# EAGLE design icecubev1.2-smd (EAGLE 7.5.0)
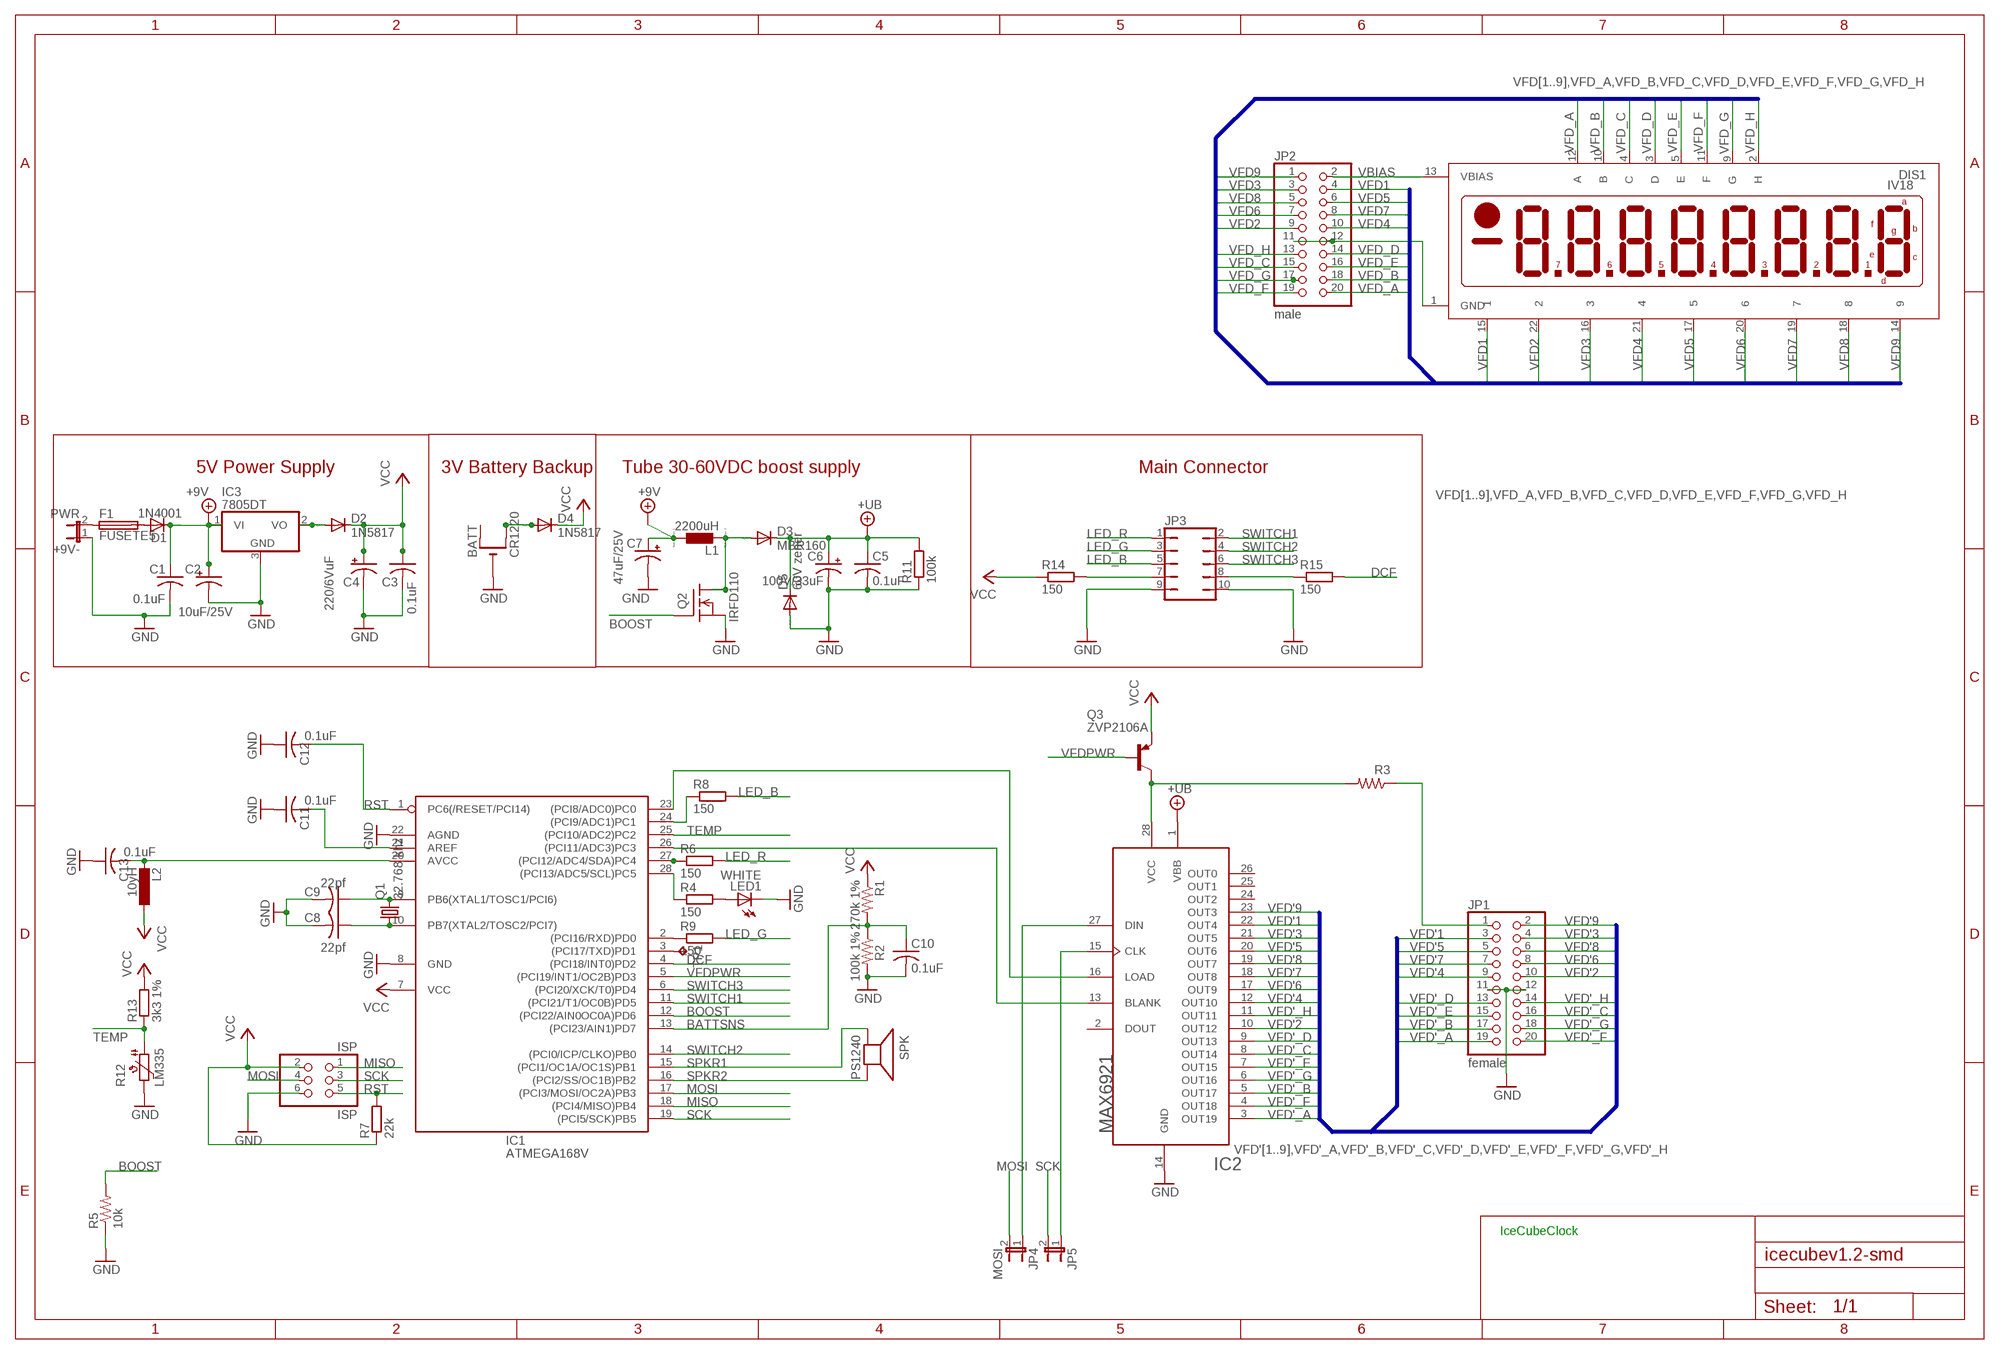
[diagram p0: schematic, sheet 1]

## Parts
+9V-  PWR  JP1E  [JP1]
BATT  CR1220  CR1220SMT  [CR1220-SMD]
C1  0.1uF  C-USC1206  [C1206]
C2  10uF/25V  CPOL-US153CLV-0405  [153CLV-0405]
C3  0.1uF  C-USC1206  [C1206]
C4  220/6VuF  CPOL-US153CLV-0405  [153CLV-0405]
C5  0.1uF  C-USC1206  [C1206]
C6  100V/33uF  CPOL-US153CLV-0405  [153CLV-0405]
C7  47uF/25V  CPOL-US153CLV-0405  [153CLV-0405]
C8  22pf  C-USC1206  [C1206]
C9  22pf  C-USC1206  [C1206]
C10  0.1uF  C-USC1206  [C1206]
C11  0.1uF  C-USC1206  [C1206]
C12  0.1uF  C-USC1206  [C1206]
C13  0.1uF  C-USC1206  [C1206]
D1  1N4001  DIODE-SOD80C  [SOD80C]
D2  1N5817  DIODE-SOD80C  [SOD80C]
D3  MBR160  DIODE-SOD80C  [SOD80C]
D4  1N5817  DIODE-SOD80C  [SOD80C]
D5  60V zener  DIODE-SOD80C  [SOD80C]
DIS1  IV18  [IV18]
F1  FUSETE5  [TE5]
IC1  ATMEGA168V  ATMEGA168PROUND  [DIL28/3]
IC2  MAX6921  [PLCC-S28]
IC3  7805DT  [TO252]
ISP  ISP  PINHD-2X3  [2X03]
JP1  female  PINHD-2X10  [2X10]
JP2  male  PINHD-2X10  [2X10]
JP3  JP5Q  [JP5Q]
JP4  MOSI  JP1E  [JP1]
JP5  JP1E  [JP1]
L1  2200uH  LL5650M  [L5650M]
L2  10yH  L-EUL4035M  [L4035M]
LED1  WHITE  LED5MM  [LED5MM]
Q1  32.768 khz  CRYTALTC26V  [TC26V]
Q2  IRFD110  [DIL04]
Q3  ZVP2106A  BC808-25-PNP-SOT23-BEC  [SOT23-BEC]
R1  270k 1%  R-US_M1206  [M1206]
R2  100k 1%  R-US_M1206  [M1206]
R3  22  R-US_M1206  [M1206]
R4  150  R-EU_M1206  [M1206]
R5  10k  R-US_R1206  [R1206]
R6  150  R-EU_M1206  [M1206]
R7  22k  R-EU_R1206  [R1206]
R8  150  R-EU_M1206  [M1206]
R9  150  R-EU_M1206  [M1206]
R11  100k  R-EU_R1206  [R1206]
R12  LM335  PTC-SOD70  [SOD70]
R13  3k3 1%  R-EU_M1206  [M1206]
R14  150  R-EU_R1206  [R1206]
R15  150  R-EU_R1206  [R1206]
SPK  PS1240  SPEAKER/PS12  [PS12]
TP1  TPB2,54  [B2,54]

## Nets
+9V: C1.1 C2.+ C7.+ D1.C IC3.1(VI) L1.1
+UB: C5.1 C6.+ D3.C D5.C IC2.1(VBB) R11.2
BATTSNS: C10.1 IC1.13((PCI23/AIN1)PD7) R1.2 R2.1
BLANK: IC1.26((PCI11/ADC3)PC3) IC2.13(BLANK)
BOOST: IC1.12((PCI22/AIN0OC0A)PD6) Q2.3(G) R5.2
DCF: IC1.4((PCI18/INT0)PD2) R15.2
GND: +9V-.1 BATT.- C1.2 C2.- C3.2 C4.- C5.2 C6.- C7.- C8.2 C9.2 C10.2 C11.1 C12.1 C13.1 D5.A DIS1.1(GND) IC1.8(GND) IC1.22(AGND) IC2.14(GND) IC3.3(GND) ISP.6 JP1.11 JP1.12 JP2.11 JP2.12 JP3.9 JP3.10 LED1.K(C) Q2.4(S) R2.2 R5.1 R11.1 R12.2
LED_B: JP3.5 R8.2
LED_G: JP3.3 R9.2
LED_R: JP3.1 R6.2
LOAD: IC1.23((PCI8/ADC0)PC0) IC2.16(LOAD)
MISO: IC1.18((PCI4/MISO)PB4) ISP.1
MOSI: IC1.17((PCI3/MOSI/OC2A)PB3) ISP.4 JP4.2
N$1: C9.1 IC1.9(PB6(XTAL1/TOSC1/PCI6)) Q1.2
N$2: D3.A L1.2 Q2.1(D) Q2.2(D1)
N$3: C8.1 IC1.10(PB7(XTAL2/TOSC2/PCI7)) Q1.1
N$4: +9V-.2 F1.1
N$5: D1.A F1.2
N$6: IC1.27((PCI12/ADC4/SDA)PC4) R6.1
N$7: IC1.28((PCI13/ADC5/SCL)PC5) R4.1
N$8: IC1.24((PCI9/ADC1)PC1) R8.1
N$9: IC1.2((PCI16/RXD)PD0) R9.1
N$10: BATT.+$2(+1) D4.A
N$11: JP3.8 R15.1
N$12: JP3.7 R14.2
N$13: LED1.A R4.2
N$14: C11.2 IC1.21(AREF)
N$15: C13.2 IC1.20(AVCC) L2.2
N$16: IC2.27(DIN) JP4.1
N$17: IC2.15(CLK) JP5.1
N$18: IC1.3((PCI17/TXD)PD1) TP1.TP
N$34: JP1.1 R3.1
N$39: IC2.28(VCC) Q3.C R3.2
N$53: D2.A IC3.2(VO)
RST: C12.2 IC1.1(PC6(/RESET/PCI14)) ISP.5 R7.2
SCK: IC1.19((PCI5/SCK)PB5) ISP.3 JP5.2
SPKR1: IC1.15((PCI1/OC1A/OC1S)PB1) SPK.P$1(+)
SPKR2: IC1.16((PCI2/SS/OC1B)PB2) SPK.P$2(-)
SWITCH1: IC1.11((PCI21/T1/OC0B)PD5) JP3.2
SWITCH2: IC1.14((PCI0/ICP/CLKO)PB0) JP3.4
SWITCH3: IC1.6((PCI20/XCK/T0)PD4) JP3.6
TEMP: IC1.25((PCI10/ADC2)PC2) R12.1 R13.1
VBIAS: DIS1.13(VBIAS) JP2.2
VCC: C3.1 C4.+ D2.C D4.C IC1.7(VCC) ISP.2 L2.1 Q3.E R1.1 R7.1 R13.2 R14.1
VFD1: DIS1.15 JP2.4
VFD2: DIS1.22 JP2.9
VFD3: DIS1.16 JP2.3
VFD4: DIS1.21 JP2.10
VFD5: DIS1.17 JP2.6
VFD6: DIS1.20 JP2.7
VFD7: DIS1.19 JP2.8
VFD8: DIS1.18 JP2.5
VFD9: DIS1.14 JP2.1
VFD'1: IC2.22(OUT4) JP1.3
VFD'2: IC2.10(OUT12) JP1.10
VFD'3: IC2.21(OUT5) JP1.4
VFD'4: IC2.12(OUT10) JP1.9
VFD'5: IC2.20(OUT6) JP1.5
VFD'6: IC2.17(OUT9) JP1.8
VFD'7: IC2.18(OUT8) JP1.7
VFD'8: IC2.19(OUT7) JP1.6
VFD'9: IC2.23(OUT3) JP1.2
VFD'_A: IC2.3(OUT19) JP1.19
VFD'_B: IC2.5(OUT17) JP1.17
VFD'_C: IC2.8(OUT14) JP1.16
VFD'_D: IC2.9(OUT13) JP1.13
VFD'_E: IC2.7(OUT15) JP1.15
VFD'_F: IC2.4(OUT18) JP1.20
VFD'_G: IC2.6(OUT16) JP1.18
VFD'_H: IC2.11(OUT11) JP1.14
VFD_A: DIS1.12(A) JP2.20
VFD_B: DIS1.10(B) JP2.18
VFD_C: DIS1.4(C) JP2.15
VFD_D: DIS1.3(D) JP2.14
VFD_E: DIS1.5(E) JP2.16
VFD_F: DIS1.11(F) JP2.19
VFD_G: DIS1.9(G) JP2.17
VFD_H: DIS1.2(H) JP2.13
VFDPWR: IC1.5((PCI19/INT1/OC2B)PD3) Q3.B
Unconnected: BATT.+$1(+) IC2.2(DOUT) IC2.24(OUT2) IC2.25(OUT1) IC2.26(OUT0)

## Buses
VFD[1..9],VFD_A,VFD_B,VFD_C,VFD_D,VFD_E,VFD_F,VFD_G,VFD_H
VFD'[1..9],VFD'_A,VFD'_B,VFD'_C,VFD'_D,VFD'_E,VFD'_F,VFD'_G,VFD'_H

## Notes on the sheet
- 5V Power Supply | 3V Battery Backup | Tube 30-60VDC boost supply | Main Connector
- IceCubeClock

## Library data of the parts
+9V- JP4 JP5 = jumper:JP1E: JUMPER
BATT = vfd:CR1220
C1 C3 C8 C9 C11-C13 = minimidi:C-US: CAPACITOR, American symbol
C2 C4 C7 = minimidi:CPOL-US: POLARIZED CAPACITOR, American symbol
C5 C10 = rcl-ez:C-US: CAPACITOR, American symbol
C6 = rcl-ez:CPOL-US: POLARIZED CAPACITOR, American symbol
D1-D5 = diode:DIODE-: DIODE
DIS1 = vfd:IV18: LCD DISPLAY 8-character 7 segment
F1 = fuse:FUSE: Fuse
IC1 = avr:ATMEGA168*P: MICROCONTROLLER 16 kBytes FLASH 1 kBytes SRAM 512 Bytes EEPROM USART 8-channel 10 bit ADC
IC2 = vfd:MAX6921
IC3 = linear:78*: Positive VOLTAGE REGULATOR
ISP = pinhead-ez:PINHD-2X3: PIN HEADER
JP1 JP2 = pinhead:PINHD-2X10: PIN HEADER
JP3 = jumper:JP5Q: JUMPER
L1 = eagle-ltspice:L: INDUCTOR, European symbol; SPICEMODEL: NONE; SPICEPREFIX: L
L2 = rcl:L-EU: INDUCTOR, European symbol
LED1 = led:LED: LED
Q1 = crystal:CRYTAL: CRYSTAL
Q2 = vfd:IRFD110
Q3 = transistor:*-PNP-: PNP Transistror
R1-R3 R5 = minimidi:R-US_: RESISTOR, American symbol
R4 R6 R8 R9 R13-R15 = resistor:R-EU_: RESISTOR, European symbol
R7 R11 = rcl:R-EU_: RESISTOR, European symbol
R12 = ptc-ntc:PTC-: Positive Temperature Coefficient Resistor (PTC) termistor; OC_FARNELL: unknown; OC_NEWARK: unknown
SPK = ybox2:SPEAKER: SPEAKER
TP1 = testpad:TP: Test pad

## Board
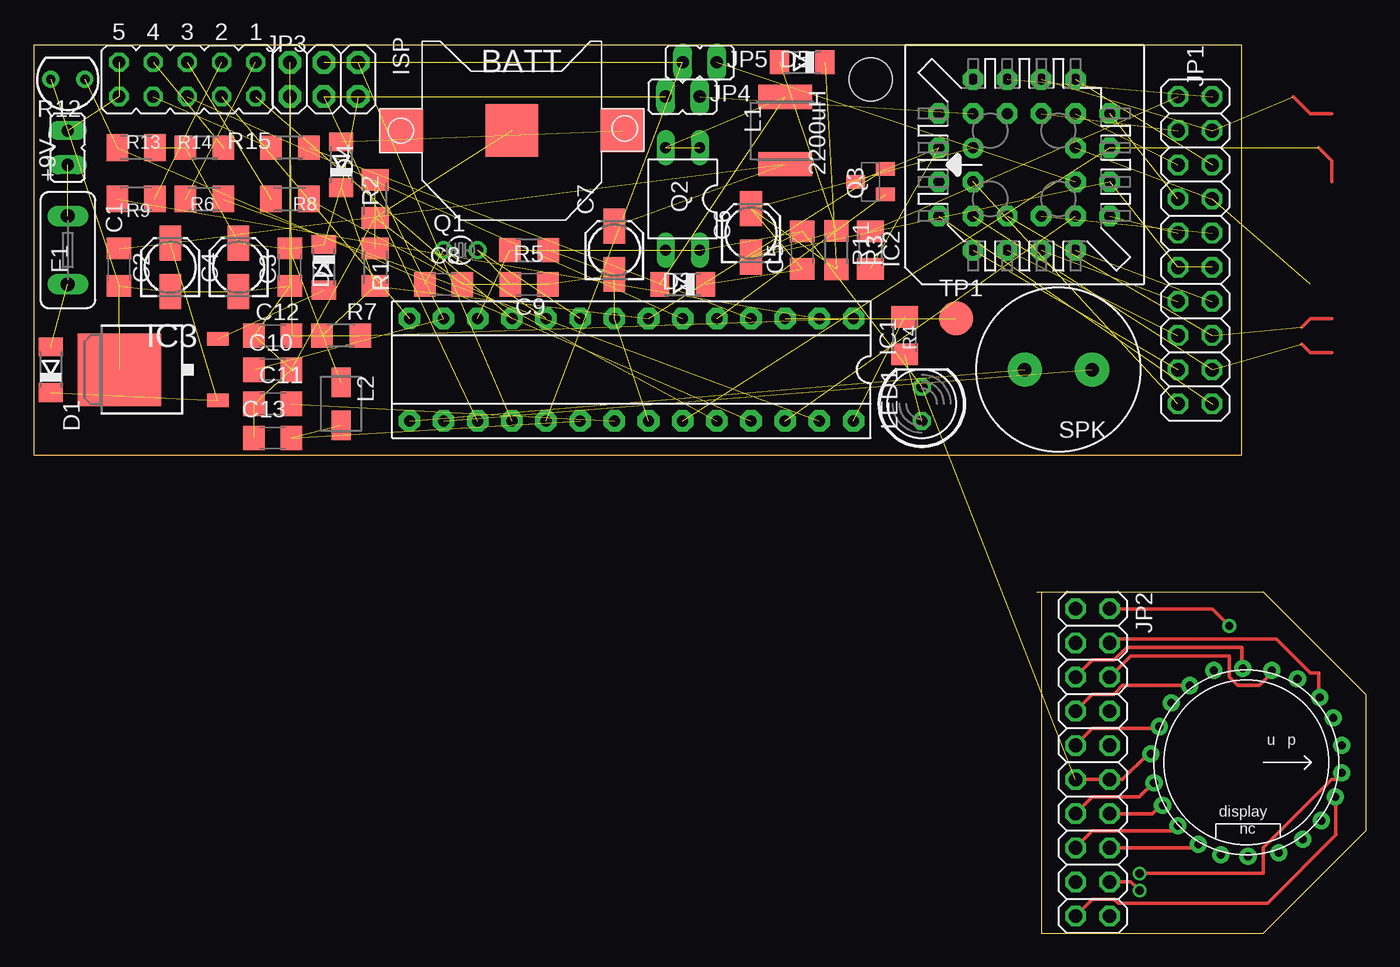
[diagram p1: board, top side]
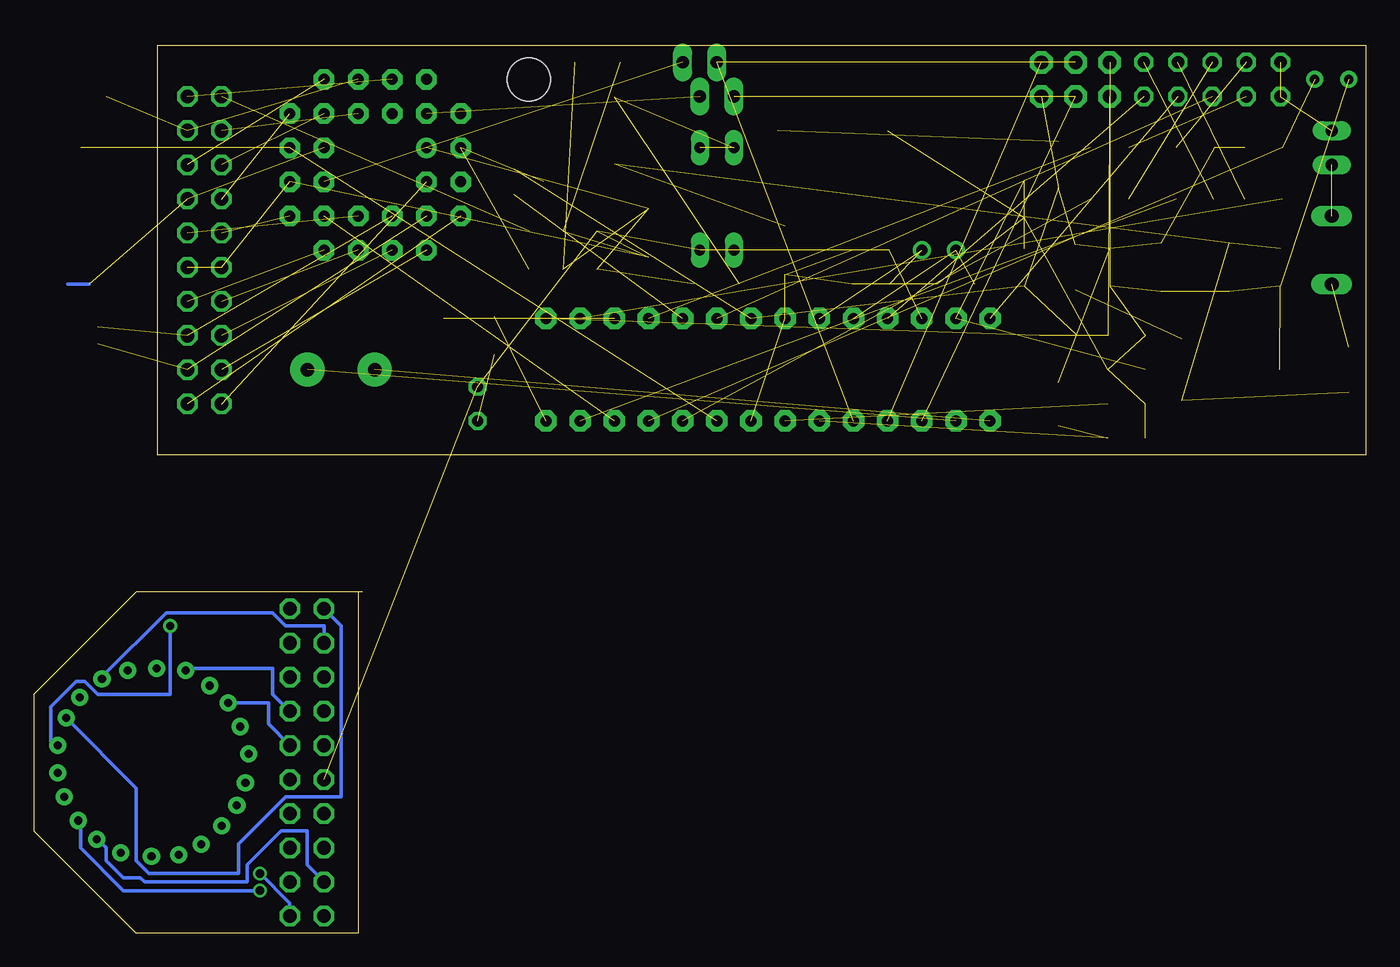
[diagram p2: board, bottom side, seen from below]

Size 99.06 x 66.03 mm. Coordinates in mm from the lower left corner, seen from the top.
Outline: 74.6,25.4 91.44,25.4 99.06,17.77 99.06,7.62
Outline: 74.93,25.39 74.93,0 91.44,0 99.06,7.61
Outline: 89.84,35.56 89.84,66.03 0,66.03 0,35.56 89.84,35.56
Copper layers (1*16): Top 0.035mm / dielectric 1.5mm / Bottom 0.035mm
Design rules "default": minimum track width 10mil, minimum drill 24mil, track to track 8mil, track to pad 8mil, pad to pad 8mil, via to via 8mil, smd to smd 8mil, copper to edge 40mil, drill to drill 8mil, minimum pad ring 10mil, minimum via ring 8mil, stop-mask expansion 4mil, vias tented up to drill 0mil, thermal gap 10mil
Holes 3.2 mm at 62.23,63.5

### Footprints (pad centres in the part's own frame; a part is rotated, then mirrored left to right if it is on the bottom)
JP1 = drill 0.914 long: 1 0,-1.27; 2 0,1.27
CR1220-SMD = smd 3.2 x 3.2: +$1 -8.2,0; +$2 8.2,0 | smd 3.9 x 3.9: - 0,0
C1206 = smd 1.6 x 1.8: 1 -1.4,0; 2 1.4,0
153CLV-0405 = smd 2.6 x 1.6: + 1.8,0; - -1.8,0
SOD80C = smd 1.4 x 1.8: A 1.7,0; C -1.7,0
IV18 = drill 0.6 pad 1.27: 1 -0.635,-7.112; 2 1.524,-6.858; 3 3.175,-6.223; 4 4.699,-5.08; 5 6.096,-3.556; 6 6.858,-1.905; 7 6.985,0.127; 8 6.731,2.413; 9 5.715,4.191; 10 4.318,5.588; 11 2.54,6.604; 12 0.762,7.112; 13 -1.27,7.112; 14 -3.302,6.477; 15 -4.826,5.461; 16 -6.223,3.81; 17 -6.858,1.905; 18 -6.985,-0.254; 19 -6.858,-2.413; 20 -5.715,-4.191; 21 -4.445,-5.588; 22 -2.667,-6.477
TE5 = drill 1.016 long: 1 -2.54,0; 2 2.54,0
DIL28/3 = drill 0.813 pad 1.6 octagon: 1 -16.51,-3.81; 2 -13.97,-3.81; 3 -11.43,-3.81; 4 -8.89,-3.81; 5 -6.35,-3.81; 6 -3.81,-3.81; 7 -1.27,-3.81; 8 1.27,-3.81; 9 3.81,-3.81; 10 6.35,-3.81; 11 8.89,-3.81; 12 11.43,-3.81; 13 13.97,-3.81; 14 16.51,-3.81; 15 16.51,3.81; 16 13.97,3.81; 17 11.43,3.81; 18 8.89,3.81; 19 6.35,3.81; 20 3.81,3.81; 21 1.27,3.81; 22 -1.27,3.81; 23 -3.81,3.81; 24 -6.35,3.81; 25 -8.89,3.81; 26 -11.43,3.81; 27 -13.97,3.81; 28 -16.51,3.81
PLCC-S28 = drill 0.813 pad 1.524: 1 1.27,3.81 | drill 0.813 pad 1.524 octagon: 2 -1.27,6.35; 3 -1.27,3.81; 4 -3.81,6.35; 5 -6.35,3.81; 6 -3.81,3.81; 7 -6.35,1.27; 8 -3.81,1.27; 9 -6.35,-1.27; 10 -3.81,-1.27; 11 -6.35,-3.81; 12 -3.81,-6.35; 13 -3.81,-3.81; 14 -1.27,-6.35; 15 -1.27,-3.81; 16 1.27,-6.35; 17 1.27,-3.81; 18 3.81,-6.35; 19 6.35,-3.81; 20 3.81,-3.81; 21 6.35,-1.27; 22 3.81,-1.27; 23 6.35,1.27; 24 3.81,1.27; 25 6.35,3.81; 26 3.81,6.35; 27 3.81,3.81; 28 1.27,6.35
TO252 = smd 1 x 1.6: 1 -2.28,-4.8; 2 2.28,-4.8 | smd 5.4 x 6.2: 3 0,2.5
2X03 = drill 1.016 pad 1.676 octagon: 1 -2.54,-1.27; 2 -2.54,1.27; 3 0,-1.27; 4 0,1.27; 5 2.54,-1.27; 6 2.54,1.27
2X10 = drill 1.016 octagon: 1 -11.43,-1.27; 2 -11.43,1.27; 3 -8.89,-1.27; 4 -8.89,1.27; 5 -6.35,-1.27; 6 -6.35,1.27; 7 -3.81,-1.27; 8 -3.81,1.27; 9 -1.27,-1.27; 10 -1.27,1.27; 11 1.27,-1.27; 12 1.27,1.27; 13 3.81,-1.27; 14 3.81,1.27; 15 6.35,-1.27; 16 6.35,1.27; 17 8.89,-1.27; 18 8.89,1.27; 19 11.43,-1.27; 20 11.43,1.27
JP5Q = drill 0.914 octagon: 1 -5.08,-1.27; 2 -5.08,1.27; 3 -2.54,-1.27; 4 -2.54,1.27; 5 0,-1.27; 6 0,1.27; 7 2.54,-1.27; 8 2.54,1.27; 9 5.08,-1.27; 10 5.08,1.27
L5650M = smd 1.8 x 4: 1 -2.5,0; 2 2.5,0
L4035M = smd 2.2 x 1.4: 1 -1.6,0; 2 1.6,0
LED5MM = drill 0.813 octagon: A -1.27,0; K 1.27,0
TC26V = drill 0.813: 1 -1.27,0; 2 1.27,0
DIL04 = drill 0.813 long: 1 -1.27,-3.81; 2 1.27,-3.81; 3 1.27,3.81; 4 -1.27,3.81
SOT23-BEC = smd 1 x 1.4: B -0.95,-1.1; C 0,1.1; E 0.95,-1.1
M1206 = smd 1.6 x 2: 1 -1.4,0; 2 1.4,0
R1206 = smd 1.6 x 1.803: 1 -1.422,0; 2 1.422,0
SOD70 = drill 0.7 pad 1.27: 1 -1.27,0; 2 1.27,0
PS12 = drill 1 pad 2.54: P$1 -2.5,0; P$2 2.5,0
B2,54 = smd 2.54 x 2.54: TP 0,0

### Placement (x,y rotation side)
+9V-  2.54,58.42 180 top
BATT  35.56,59.69 0 top
C1  6.35,49.53 270 top
C2  10.16,49.53 90 top
C3  19.05,49.53 270 top
C4  15.24,49.53 90 top
C5  57.15,50.8 90 top
C6  53.34,52.07 90 top
C7  43.18,50.8 90 top
C8  30.48,48.26 0 top
C9  36.83,48.26 0 top
C10  17.78,41.91 0 top
C11  17.78,39.37 0 top
C12  17.78,44.45 0 top
C13  17.78,36.83 0 top
D1  1.27,41.91 90 top
D2  21.59,49.53 270 top
D3  48.26,48.26 180 top
D4  22.86,57.15 90 top
D5  57.15,64.77 180 top
DIS1  90.17,12.7 270 top
F1  2.54,50.8 270 top
IC1  44.45,41.91 180 top
IC2  73.66,57.15 90 top
IC3  8.89,41.91 90 top
ISP  21.59,63.5 180 top
JP1  86.36,50.8 270 top
JP2  78.74,12.7 270 top
JP3  11.43,63.5 180 top
JP4  48.26,62.23 90 top
JP5  49.53,64.77 90 top
L1  55.88,59.69 90 top
L2  22.86,39.37 270 top
LED1  66.04,39.37 90 top
Q1  31.75,50.8 0 top
Q2  48.26,54.61 180 top
Q3  62.23,55.88 90 top
R1  25.4,49.53 90 top
R2  25.4,54.61 270 top
R3  62.23,50.8 270 top
R4  64.77,44.45 270 top
R5  36.83,50.8 180 top
R6  12.7,54.61 180 top
R7  22.86,44.45 0 top
R8  19.05,54.61 180 top
R9  7.62,54.61 0 top
R11  59.69,50.8 270 top
R12  2.54,63.5 180 top
R13  7.62,58.42 0 top
R14  12.7,58.42 0 top
R15  19.05,58.42 0 top
SPK  76.2,41.91 0 top
TP1  68.58,45.72 0 top

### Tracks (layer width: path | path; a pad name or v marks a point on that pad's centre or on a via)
+9V  (5 unrouted)
+UB  (5 unrouted)
BATTSNS  (3 unrouted)
BLANK  (1 unrouted)
BOOST  (2 unrouted)
DCF  (1 unrouted)
GND  (31 unrouted)
  Top 0.254: DIS1.1 82.87,13.34 80.96,11.43 JP2.12 JP2.11
LED_B  (1 unrouted)
LED_G  (1 unrouted)
LED_R  (1 unrouted)
LOAD  (2 unrouted)
  Top 0.254: 95.57,58.42 96.52,57.47 96.52,55.88
MISO  (1 unrouted)
MOSI  (2 unrouted)
N$1  (2 unrouted)
N$2  (3 unrouted)
N$3  (2 unrouted)
N$4  (1 unrouted)
N$5  (1 unrouted)
N$6  (1 unrouted)
N$7  (1 unrouted)
N$8  (1 unrouted)
N$9  (1 unrouted)
N$10  (1 unrouted)
N$11  (1 unrouted)
N$12  (1 unrouted)
N$13  (1 unrouted)
N$14  (1 unrouted)
N$15  (2 unrouted)
N$16  (1 unrouted)
N$17  (1 unrouted)
N$18  (1 unrouted)
N$34  (1 unrouted)
N$39  (2 unrouted)
N$53  (1 unrouted)
RST  (3 unrouted)
SCK  (2 unrouted)
SPKR1  (1 unrouted)
SPKR2  (1 unrouted)
SWITCH1  (1 unrouted)
SWITCH2  (1 unrouted)
SWITCH3  (1 unrouted)
TEMP  (2 unrouted)
VBIAS  (via drill 0.61)
  Top 0.254: v88.9,22.86 87.63,24.13 JP2.2
  Bottom 0.254: v88.9,22.86 88.9,17.78 94.3,17.78 95.25,18.73 95.89,18.73 97.79,16.83 97.79,14.29 97.47,13.97 DIS1.13
VCC  (11 unrouted)
VFD1
  Top 0.254: JP2.4 80.33,21.91 92.39,21.91 94.93,19.37 95.57,19.37 95.57,17.78 DIS1.15
VFD2
  Top 0.254: JP2.9 78.74,15.24 83.5,15.24 DIS1.22
VFD3
  Bottom 0.254: JP2.3 77.47,22.86 80.33,22.86 81.28,23.81 89.22,23.81 93.98,19.05 DIS1.16
VFD4
  Bottom 0.254: DIS1.21 81.6,17.14 81.6,15.56 JP2.10
VFD5
  Top 0.254: JP2.6 81.6,20.64 88.9,20.64 88.9,19.05 89.53,18.41 91.12,18.41 92.08,19.37 DIS1.17
VFD6
  Top 0.254: DIS1.20 80.96,18.41 80.33,17.78 78.74,17.78 JP2.7
VFD7
  Bottom 0.254: JP2.8 81.28,17.78 81.28,19.68 87.63,19.68 DIS1.19
VFD8
  Top 0.254: JP2.5 78.74,20.32 80.33,20.32 81.28,21.27 89.85,21.27 89.85,19.68 DIS1.18
VFD9
  Bottom 0.254: DIS1.14 91.44,10.79 91.44,5.4 90.49,4.45 83.82,4.45 83.82,6.67 80.33,10.16 76.2,10.16 76.2,22.86 JP2.1
VFD'1  (1 unrouted)
VFD'2  (1 unrouted)
VFD'3  (2 unrouted)
  Top 0.254: 93.66,62.23 94.93,60.96 96.52,60.96
VFD'4  (1 unrouted)
VFD'5  (1 unrouted)
VFD'6  (2 unrouted)
  Bottom 0.254: 96.52,48.26 94.93,48.26
VFD'7  (1 unrouted)
VFD'8  (1 unrouted)
VFD'9  (1 unrouted)
VFD'_A  (1 unrouted)
VFD'_B  (1 unrouted)
VFD'_C  (2 unrouted)
  Top 0.254: 94.3,45.08 94.93,45.72 96.52,45.72
VFD'_D  (1 unrouted)
VFD'_E  (1 unrouted)
VFD'_F  (1 unrouted)
VFD'_G  (2 unrouted)
  Top 0.254: 94.3,43.81 94.93,43.18 96.52,43.18
VFD'_H  (1 unrouted)
VFD_A  (via drill 0.61)
  Top 0.254: v82.23,4.45 91.44,4.45 91.44,6.35 96.52,11.43 96.84,11.43 97.16,11.75 DIS1.12
  Bottom 0.254: v82.23,4.45 80.01,2.22 JP2.20
VFD_B  (via drill 0.61)
  Top 0.254: v82.23,3.18 81.6,3.81 JP2.18
  Bottom 0.254: v82.23,3.18 92.39,3.18 95.57,6.35 95.57,8.25 DIS1.10
VFD_C
  Top 0.254: JP2.15 78.74,7.62 84.77,7.62 85.09,7.94 DIS1.4
VFD_D
  Top 0.254: JP2.14 83.19,8.89 83.82,9.52 DIS1.3
VFD_E
  Top 0.254: JP2.16 86.36,6.35 DIS1.5
VFD_F
  Top 0.254: JP2.19 78.74,2.54 80.33,2.54 80.64,2.22 91.76,2.22 96.84,7.3 96.84,10.16 DIS1.11
VFD_G
  Bottom 0.254: JP2.17 78.74,5.08 78.74,7.62 80.64,7.62 83.19,5.08 83.19,3.81 90.81,3.81 91.12,4.13 92.39,4.13 93.66,5.4 93.66,6.35 94.3,6.98 DIS1.9
VFD_H
  Top 0.254: JP2.13 78.74,10.16 82.23,10.16 83.19,11.11 DIS1.2
VFDPWR  (1 unrouted)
